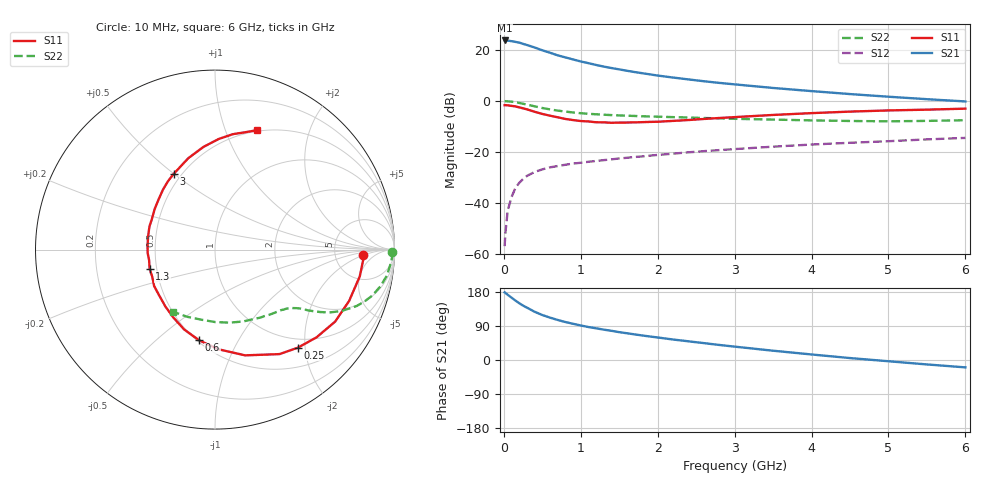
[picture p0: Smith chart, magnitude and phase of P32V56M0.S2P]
! SIEMENS Small Signal Semiconductors
! BFP181
! Si NPN RF Bipolar Junction Transistor in SOT143
! VCE = 2.5 V  IC = 6 mA
! Common Emitter S-Parameters:  March  1996
# GHz  S  MA  R  50
!  f  S11  S21  S12  S22
! GHz  MAG  ANG  MAG  ANG  MAG  ANG  MAG  ANG
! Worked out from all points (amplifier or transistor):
!   36 points, 10 MHz to 6 GHz, reference 50 ohm
!   highest |S21| = 23.8 dB at 10 MHz (marker M1)
!   |S21| within 3 dB of that: start of sweep to 421.2 MHz
!   unconditionally stable (mu >= 1): 1.504 GHz to end of sweep
!   at 250 MHz: K = 0.25, MSG = 26.6 dB, |S12| = -30.7 dB
!   at 1.4 GHz: K = 0.98, MSG = 17.9 dB, |S12| = -23.0 dB
!   at 6 GHz: K = 1.04, MAG = 6.0 dB, |S12| = -14.5 dB
!   S11 on the Smith chart (normalised r, x): 10 MHz: 10, -2; 250 MHz: 0.83, -1.86; 600 MHz: 0.51, -0.70; 1.3 GHz: 0.46, -0.11; 3 GHz: 0.45, +0.50; 6 GHz: 0.49, +1.29
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0.01  0.8248 -2.2  15.43 178.4  0.0014 82.9  0.9884 -0.7
0.05  0.8202 -10.5  15.38 172.1  0.007 85.2  0.9825 -4.4
0.1  0.8002 -20.9  14.93 164.5  0.0129 76.0  0.9687 -8.6
0.15  0.7805 -30.9  14.47 156.9  0.0194 73.2  0.944 -12.5
0.2  0.7477 -40.8  14 149.9  0.0246 69.2  0.9142 -16.2
0.25  0.7158 -49.7  13.22 143.5  0.0292 65.3  0.88 -19.3
0.3  0.6843 -58.3  12.56 138.2  0.0336 61.1  0.8483 -21.8
0.4  0.6127 -74.1  11.22 127.3  0.0402 55.8  0.7835 -25.9
0.5  0.5552 -88.2  9.887 118.7  0.0452 51.3  0.7272 -28.8
0.6  0.513 -99.9  8.855 111.8  0.0495 48.9  0.6811 -30.7
0.7  0.4771 -111.1  7.871 105.7  0.0526 46.4  0.6455 -32.1
0.8  0.4432 -121.8  7.169 100.2  0.0557 45.3  0.6179 -33.2
0.9  0.4207 -131.0  6.535 95.5  0.0588 43.9  0.5932 -34.0
1.1  0.3952 -149.1  5.518 87.0  0.0638 42.9  0.559 -35.7
1.3  0.3796 -163.7  4.721 80.1  0.0687 42.1  0.5361 -37.4
1.7  0.3791 169.9  3.696 67.6  0.0792 41.3  0.5066 -41.4
2.2  0.4052 146.0  2.879 54.1  0.092 39.9  0.4809 -47.6
3  0.4807 118.6  2.116 35.3  0.1131 36.1  0.4455 -59.7
3.5  0.5305 106.3  1.799 24.5  0.1263 33.4  0.43 -68.7
4.5  0.6171 88.0  1.364 5.1  0.1506 26.7  0.4037 -89.9
5.5  0.674 75.8  1.082 -11.7  0.1755 20.6  0.4052 -112.5
6  0.7053 70.6  0.977 -19.5  0.1878 16.8  0.4177 -124.0
